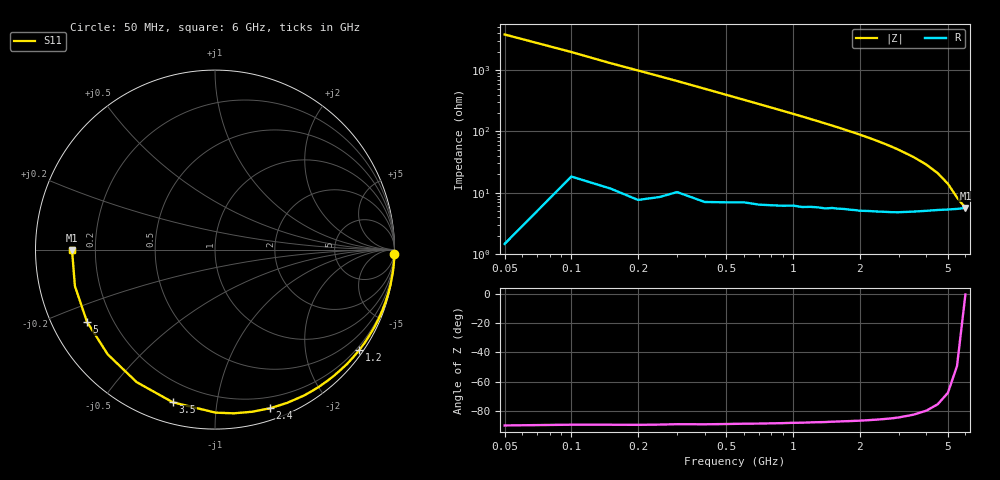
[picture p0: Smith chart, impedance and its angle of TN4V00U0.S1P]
! SIEMENS Discrete & RF Semiconductors
! BAS70-07W
! Si Schottky Diode in SOT343
! VR = 4 V
! S-Parameters:  February  1997
# GHz  S  MA  R  50
!  f  S11
! GHz  MAG  ANG
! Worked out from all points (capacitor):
!   34 points, 50 MHz to 6 GHz, reference 50 ohm
!   read as one part to ground: C = 815 fF near 50 MHz
!   lowest |Z| = 5.66 ohm at 6 GHz (marker M1)
!   S11 on the Smith chart (normalised r, x): 50 MHz: 0, -76; 1.2 GHz: 0.12, -3.19; 2.4 GHz: 0.10, -1.40; 3.5 GHz: 0.10, -0.76; 5 GHz: 0.11, -0.26; 6 GHz: 0.11, -0.00
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0.05  1 -1.5
0.2  0.9992 -5.8
0.4  0.9972 -11.5
0.5  0.9956 -14.4
0.6  0.9937 -17.3
0.7  0.9922 -20.2
0.8  0.99 -23.1
0.9  0.9877 -26.0
1  0.9847 -28.9
1.1  0.9826 -31.8
1.2  0.9792 -34.8
1.3  0.9762 -37.7
1.4  0.9736 -40.7
1.6  0.9662 -46.6
1.8  0.9591 -52.7
1.9  0.9556 -55.6
2  0.9523 -58.7
2.2  0.9438 -64.8
2.4  0.9355 -71.0
2.6  0.9267 -77.2
2.8  0.9181 -83.5
3  0.9084 -89.8
3.5  0.8826 -105.4
4  0.8578 -120.6
4.5  0.8355 -135.7
5  0.8188 -150.6
5.5  0.8066 -165.4
6  0.7967 -179.9
